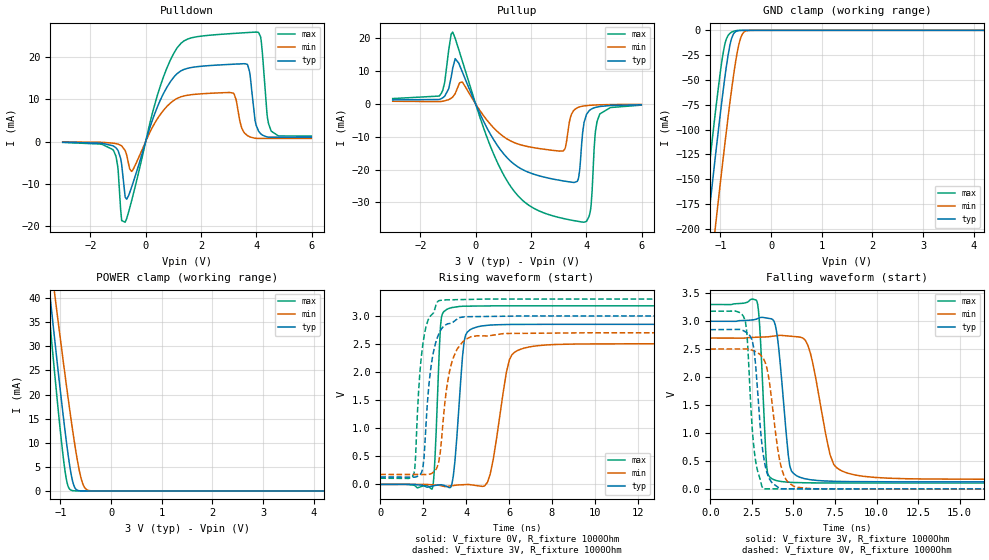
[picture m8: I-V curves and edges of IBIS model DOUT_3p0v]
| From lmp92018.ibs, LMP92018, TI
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|   Model
[Model]   DOUT_3p0v
Model_type   3-state
Polarity   Non-Inverting
Vmeas = 1.5
Vref = 0
Cref = 1pF
Rref = 1000000
|   typ   min   max
C_comp   0.5310pF   0.5030pF   0.6389pF
[Voltage Range]   3   2.7   3.3
[Temperature Range]   27   125   -40
[Pullup Reference]   3   2.7   3.3
[Pulldown Reference]   0   0   0
[Power Clamp Reference]   3   2.7   3.3
[GND Clamp Reference]   0   0   0
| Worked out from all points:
|   slope of the pulldown table from 0 to 0.45 V, typ, clamps not added: 52.1 ohm
|   slope of the pullup table from 0 to 0.45 V, typ, clamps not added: 56.7 ohm
|   GND clamp passes 1 mA (typ) near -0.69 V on its own axis
|   POWER clamp passes 1 mA (typ) near -0.73 V on its own axis
|   falling waveform, V_fixture 3V, R_fixture 1000Ohm: 20-80 % time 514ps typ, 954ps min, 303ps max; typ from 3 V to 0.131 V
|   rising waveform, V_fixture 0V, R_fixture 1000Ohm: 20-80 % time 321ps typ, 594ps min, 201ps max; typ from 0 V to 2.85 V
|   rising waveform, V_fixture 3V, R_fixture 1000Ohm: 20-80 % time 444ps typ, 527ps min, 379ps max; typ from 0.131 V to 3 V
|   falling waveform, V_fixture 0V, R_fixture 1000Ohm: 20-80 % time 507ps typ, 678ps min, 410ps max; typ from 2.85 V to 0 V
[Pulldown]
|   Voltage   I(typ)   I(min)   I(max)
-3V       -145.3uA   -78.39uA   -205.6uA
-1.191V   -981.5uA   -368.8uA   -1.893mA
-903mV    -4.039mA   -883.7uA   -16.33mA
-741mV    -13.21mA   -2.122mA   -19.16mA
-489mV    -10.45mA   -6.984mA   -13.57mA
1.131V    16.09mA    10.23mA    22.19mA
3.165V    18.37mA    11.52mA    25.68mA
3.669V    18.37mA    1.472mA    25.89mA
3.993V    3.923mA    752.7uA    26.01mA
4.173V    1.777mA    735.7uA    24.19mA
4.533V    1.032mA    735.9uA    2.617mA
5.991V    1.033mA    736.6uA    1.312mA
[GND Clamp]
|   Voltage   I(typ)   I(min)   I(max)
-3V       -1.048A    -1.117A    -1.006A
-1.353V   -244.8mA   -316.7mA   -199.4mA
-1.335V   -236.3mA   -308.2mA   -190.9mA
-1.191V   -168.9mA   -240.6mA   -123.7mA
-1.083V   -119.7mA   -190.7mA   -75.5mA
-921mV    -50.87mA   -118.3mA   -15.97mA
-813mV    -15.12mA   -73.06mA   -3.104mA
-741mV    -3.527mA   -45.63mA   -925.1uA
-669mV    -637uA     -22.53mA   -172.3uA
-597mV    -107.9uA   -7.262mA   -21.32uA
-453mV    -2.079uA   -203.5uA   0A
5.991V    0A         0A         0A
[Pullup]
|   Voltage   I(typ)   I(min)   I(max)
-3V       1.262mA    841.7uA    1.662mA
-1.317V   1.381mA    734.6uA    2.429mA
-831mV    10.88mA    2.133mA    21.92mA
645mV     -10.8mA    -7.208mA   -15.14mA
1.905V    -20.78mA   -12.99mA   -30.74mA
3.165V    -23.42mA   -14.29mA   -34.87mA
3.669V    -23.58mA   -1.157mA   -35.7mA
3.921V    -5.564mA   -574.4uA   -36mA
4.155V    -1.694mA   -372.7uA   -32.25mA
4.317V    -1.074mA   -295uA     -9.725mA
4.479V    -769.8uA   -242uA     -3.233mA
5.991V    -226.5uA   -119.5uA   -337.9uA
[POWER Clamp]
|   Voltage   I(typ)   I(min)   I(max)
-3V       220.5mA    201.8mA    243.9mA
-1.263V   46.23mA    53.62mA    41.36mA
-1.245V   44.44mA    52.08mA    39.29mA
-1.191V   39.08mA    47.48mA    33.12mA
-1.101V   30.27mA    39.87mA    23.04mA
-903mV    11.99mA    23.61mA    3.718mA
-849mV    7.601mA    19.36mA    977.2uA
-795mV    3.871mA    15.25mA    175.5uA
-723mV    832.1uA    10.08mA    24.97uA
-597mV    14.93uA    2.85mA     0A
-435mV    0A         80.48uA    0A
5.991V    0A         0A         0A
[Ramp]
R_load = 1000
|   typ   min   max
dV/dt_r   1.70995/3.20853e-10   1.50219/5.93784e-10   1.9077/2.00577e-10
dV/dt_f   1.72123/5.13769e-10   1.51403/9.54388e-10   1.91411/3.02542e-10
[Falling Waveform]
V_fixture = 3V
V_fixture_min = 2.7V
V_fixture_max = 3.3V
R_fixture = 1000Ohm
C_fixture = 0F
|   Time   V(typ)   V(min)   V(max)
0s        3V         2.7V       3.3V
2.809ns   3.043V     2.715V     3.355V
3.45ns    3.055V     2.722V     281.1mV
3.912ns   2.931V     2.739V     159.7mV
4.353ns   1.747V     2.746V     133.3mV
4.988ns   285.8mV    2.729V     119.2mV
5.878ns   176.5mV    2.566V     112.9mV
7.433ns   140.7mV    436.6mV    110.9mV
9.917ns   132.9mV    209.3mV    109.9mV
100ns     131.3mV    176.6mV    109.8mV
[Rising Waveform]
V_fixture = 0V
V_fixture_min = 0V
V_fixture_max = 0V
R_fixture = 1000Ohm
C_fixture = 0F
|   Time   V(typ)   V(min)   V(max)
0s        580.4nV    -13.75nV   -4.778uV
2.424ns   -30.43mV   -7.343mV   -73.74mV
2.85ns    -6.891mV   -25.83mV   2.974V
3.332ns   -3.512mV   -24.79mV   3.148V
3.701ns   1.575V     -9.184mV   3.169V
4.19ns    2.755V     -5.628mV   3.174V
5.123ns   2.836V     183.5mV    3.178V
6.145ns   2.848V     2.313V     3.179V
7.778ns   2.85V      2.484V     3.179V
100ns     2.85V      2.504V     3.179V
[Rising Waveform]
V_fixture = 3V
V_fixture_min = 2.7V
V_fixture_max = 3.3V
R_fixture = 1000Ohm
C_fixture = 0F
|   Time   V(typ)   V(min)   V(max)
0s        131.3mV    176.7mV    109.8mV
1.572ns   129mV      175.5mV    197.9mV
1.93ns    217.7mV    175.3mV    2.328V
2.401ns   2.19V      196.5mV    3.023V
2.71ns    2.662V     370.5mV    3.266V
2.94ns    2.811V     1.18V      3.284V
3.216ns   2.864V     1.989V     3.287V
3.599ns   2.949V     2.42V      3.29V
5.878ns   2.995V     2.687V     3.3V
100ns     3V         2.7V       3.3V
[Falling Waveform]
|Gnd
V_fixture = 0V
V_fixture_min = 0V
V_fixture_max = 0V
R_fixture = 1000Ohm
C_fixture = 0F
|   Time   V(typ)   V(min)   V(max)
0s        2.85V      2.504V     3.179V
2.087ns   2.816V     2.505V     3.021V
2.21ns    2.795V     2.505V     2.746V
2.49ns    2.679V     2.486V     1.229V
2.651ns   2.437V     2.467V     670.5mV
3.249ns   508.5mV    2.301V     5.385mV
3.665ns   132.4mV    1.662V     5.362mV
4.4ns     6.079mV    268.6mV    5.321mV
6.145ns   5.969mV    6.912mV    5.223mV
100ns     591.7nV    76.3nV     -4.848uV
